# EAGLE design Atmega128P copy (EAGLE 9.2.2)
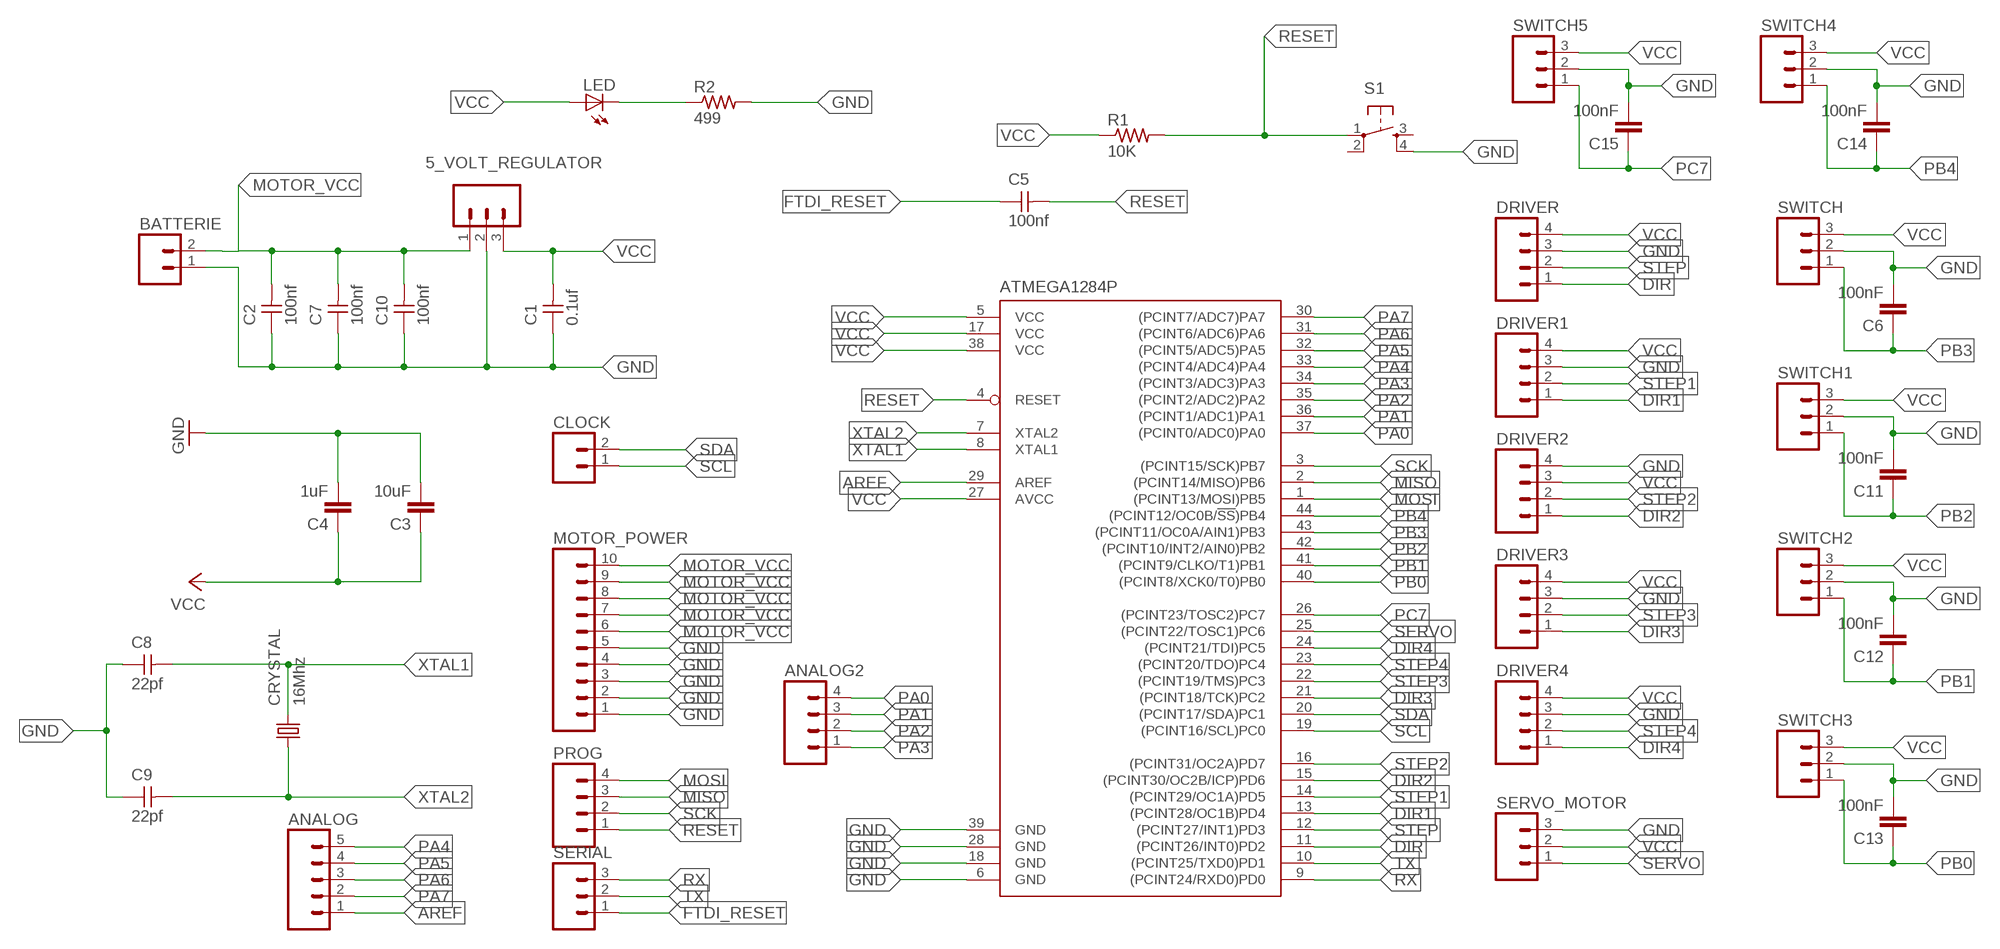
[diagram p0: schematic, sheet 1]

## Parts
5_VOLT_REGULATOR  M03  [03P]
ANALOG  M05  [05P]
ANALOG2  M04  [04P]
ATMEGA1284P  ATMEGA644A  [TQFP44]
BATTERIE  M02  [02P]
C1  0.1uf  UNPOLARIZED_CAPACITOR1206  [1206]
C2  100nf  UNPOLARIZED_CAPACITOR1206  [1206]
C3  10uF  CAP1206  [1206]
C4  1uF  CAP1206  [1206]
C5  100nf  UNPOLARIZED_CAPACITOR1206  [1206]
C6  100nF  CAP1206  [1206]
C7  100nf  UNPOLARIZED_CAPACITOR1206  [1206]
C8  22pf  UNPOLARIZED_CAPACITOR1206  [1206]
C9  22pf  UNPOLARIZED_CAPACITOR1206  [1206]
C10  100nf  UNPOLARIZED_CAPACITOR1206  [1206]
C11  100nF  CAP1206  [1206]
C12  100nF  CAP1206  [1206]
C13  100nF  CAP1206  [1206]
C14  100nF  CAP1206  [1206]
C15  100nF  CAP1206  [1206]
CLOCK  M02  [02P]
CRYSTAL  16Mhz  KX-12B  [6.0X3.5_2]
DRIVER  M04  [04P]
DRIVER1  M04  [04P]
DRIVER2  M04  [04P]
DRIVER3  M04  [04P]
DRIVER4  M04  [04P]
LED  LED1206  [1206]
MOTOR_POWER  M10  [10P]
PROG  M04  [04P]
R1  10K  RESISTOR1206  [1206]
R2  499  RESISTOR1206  [1206]
S1  6MM_SWITCH6MM_SWITCH  [6MM_SWITCH]
SERIAL  M03  [03P]
SERVO_MOTOR  M03  [03P]
SWITCH  M03  [03P]
SWITCH1  M03  [03P]
SWITCH2  M03  [03P]
SWITCH3  M03  [03P]
SWITCH4  M03  [03P]
SWITCH5  M03  [03P]

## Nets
AREF: ANALOG.1 ATMEGA1284P.29(AREF)
DIR: ATMEGA1284P.11((PCINT26/INT0)PD2) DRIVER.1
DIR1: ATMEGA1284P.13((PCINT28/OC1B)PD4) DRIVER1.1
DIR2: ATMEGA1284P.15((PCINT30/OC2B/ICP)PD6) DRIVER2.1
DIR3: ATMEGA1284P.21((PCINT18/TCK)PC2) DRIVER3.1
DIR4: ATMEGA1284P.24((PCINT21/TDI)PC5) DRIVER4.1
FTDI_RESET: C5.1 SERIAL.1
GND: 5_VOLT_REGULATOR.2 ATMEGA1284P.6(GND) ATMEGA1284P.18(GND) ATMEGA1284P.28(GND) ATMEGA1284P.39(GND) BATTERIE.1 C1.1 C2.1 C3.2 C4.2 C6.2 C7.1 C8.1 C9.1 C10.1 C11.2 C12.2 C13.2 C14.2 C15.2 DRIVER1.3 DRIVER2.4 DRIVER3.3 DRIVER4.3 DRIVER.3 MOTOR_POWER.1 MOTOR_POWER.2 MOTOR_POWER.3 MOTOR_POWER.4 MOTOR_POWER.5 R2.2 S1.4(S1) SERVO_MOTOR.3 SWITCH1.2 SWITCH2.2 SWITCH3.2 SWITCH4.2 SWITCH5.2 SWITCH.2
MISO: ATMEGA1284P.2((PCINT14/MISO)PB6) PROG.3
MOSI: ATMEGA1284P.1((PCINT13/MOSI)PB5) PROG.4
MOTOR_VCC: 5_VOLT_REGULATOR.1 BATTERIE.2 C2.2 C7.2 C10.2 MOTOR_POWER.6 MOTOR_POWER.7 MOTOR_POWER.8 MOTOR_POWER.9 MOTOR_POWER.10
N$1: LED.2(C) R2.1
PA0: ANALOG2.4 ATMEGA1284P.37((PCINT0/ADC0)PA0)
PA1: ANALOG2.3 ATMEGA1284P.36((PCINT1/ADC1)PA1)
PA2: ANALOG2.2 ATMEGA1284P.35((PCINT2/ADC2)PA2)
PA3: ANALOG2.1 ATMEGA1284P.34((PCINT3/ADC3)PA3)
PA4: ANALOG.5 ATMEGA1284P.33((PCINT4/ADC4)PA4)
PA5: ANALOG.4 ATMEGA1284P.32((PCINT5/ADC5)PA5)
PA6: ANALOG.3 ATMEGA1284P.31((PCINT6/ADC6)PA6)
PA7: ANALOG.2 ATMEGA1284P.30((PCINT7/ADC7)PA7)
PB0: ATMEGA1284P.40((PCINT8/XCK0/T0)PB0) C13.1 SWITCH3.1
PB1: ATMEGA1284P.41((PCINT9/CLKO/T1)PB1) C12.1 SWITCH2.1
PB2: ATMEGA1284P.42((PCINT10/INT2/AIN0)PB2) C11.1 SWITCH1.1
PB3: ATMEGA1284P.43((PCINT11/OC0A/AIN1)PB3) C6.1 SWITCH.1
PB4: ATMEGA1284P.44((PCINT12/OC0B/!SS!)PB4) C14.1 SWITCH4.1
PC7: ATMEGA1284P.26((PCINT23/TOSC2)PC7) C15.1 SWITCH5.1
RESET: ATMEGA1284P.4(RESET) C5.2 PROG.1 R1.2 S1.1(P)
RX: ATMEGA1284P.9((PCINT24/RXD0)PD0) SERIAL.3
SCK: ATMEGA1284P.3((PCINT15/SCK)PB7) PROG.2
SCL: ATMEGA1284P.19((PCINT16/SCL)PC0) CLOCK.1
SDA: ATMEGA1284P.20((PCINT17/SDA)PC1) CLOCK.2
SERVO: ATMEGA1284P.25((PCINT22/TOSC1)PC6) SERVO_MOTOR.1
STEP: ATMEGA1284P.12((PCINT27/INT1)PD3) DRIVER.2
STEP1: ATMEGA1284P.14((PCINT29/OC1A)PD5) DRIVER1.2
STEP2: ATMEGA1284P.16((PCINT31/OC2A)PD7) DRIVER2.2
STEP3: ATMEGA1284P.22((PCINT19/TMS)PC3) DRIVER3.2
STEP4: ATMEGA1284P.23((PCINT20/TDO)PC4) DRIVER4.2
TX: ATMEGA1284P.10((PCINT25/TXD0)PD1) SERIAL.2
VCC: 5_VOLT_REGULATOR.3 ATMEGA1284P.5(VCC) ATMEGA1284P.17(VCC) ATMEGA1284P.27(AVCC) ATMEGA1284P.38(VCC) C1.2 C3.1 C4.1 DRIVER1.4 DRIVER2.3 DRIVER3.4 DRIVER4.4 DRIVER.4 LED.1(A) R1.1 SERVO_MOTOR.2 SWITCH1.3 SWITCH2.3 SWITCH3.3 SWITCH4.3 SWITCH5.3 SWITCH.3
XTAL1: ATMEGA1284P.8(XTAL1) C8.2 CRYSTAL.2
XTAL2: ATMEGA1284P.7(XTAL2) C9.2 CRYSTAL.1
Unconnected: S1.2(P1) S1.3(S)

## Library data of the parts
5_VOLT_REGULATOR SERIAL SERVO_MOTOR SWITCH SWITCH1-SWITCH5 = con-amp-quick:M03: AMP QUICK CONNECTOR; OC_FARNELL: unknown; OC_NEWARK: unknown
ANALOG = con-amp-quick:M05: AMP QUICK CONNECTOR; OC_FARNELL: unknown; OC_NEWARK: unknown
ANALOG2 DRIVER DRIVER1-DRIVER4 PROG = con-amp-quick:M04: AMP QUICK CONNECTOR; OC_FARNELL: unknown; OC_NEWARK: unknown
ATMEGA1284P = atmel:ATMEGA644: 8-bit Microcontroller with 64K Bytes In-System Programmable Flash Source: http://www.atmel.com/dyn/resources/prod_documents/doc2593.pdf; MPN: ATMEGA644PV-10AU; OC_FARNELL: 1455123; OC_NEWARK: 58M3748
BATTERIE CLOCK = con-amp-quick:M02: AMP QUICK CONNECTOR; OC_FARNELL: unknown; OC_NEWARK: unknown
C1 C2 C5 C7-C10 = FAB_Hello:UNPOLARIZED_CAPACITOR: unpolarized_capacitor
C3 C4 C6 C11-C15 = 01_SparkFun:CAP: Capacitor
CRYSTAL = crystal-geyer_V1_0:KX
LED = FAB_Hello:LED
MOTOR_POWER = con-amp-quick:M10: AMP QUICK CONNECTOR; OC_FARNELL: unknown; OC_NEWARK: unknown
R1 R2 = FAB_Hello:RESISTOR
S1 = FAB_Hello:6MM_SWITCH: OMRON SWITCH

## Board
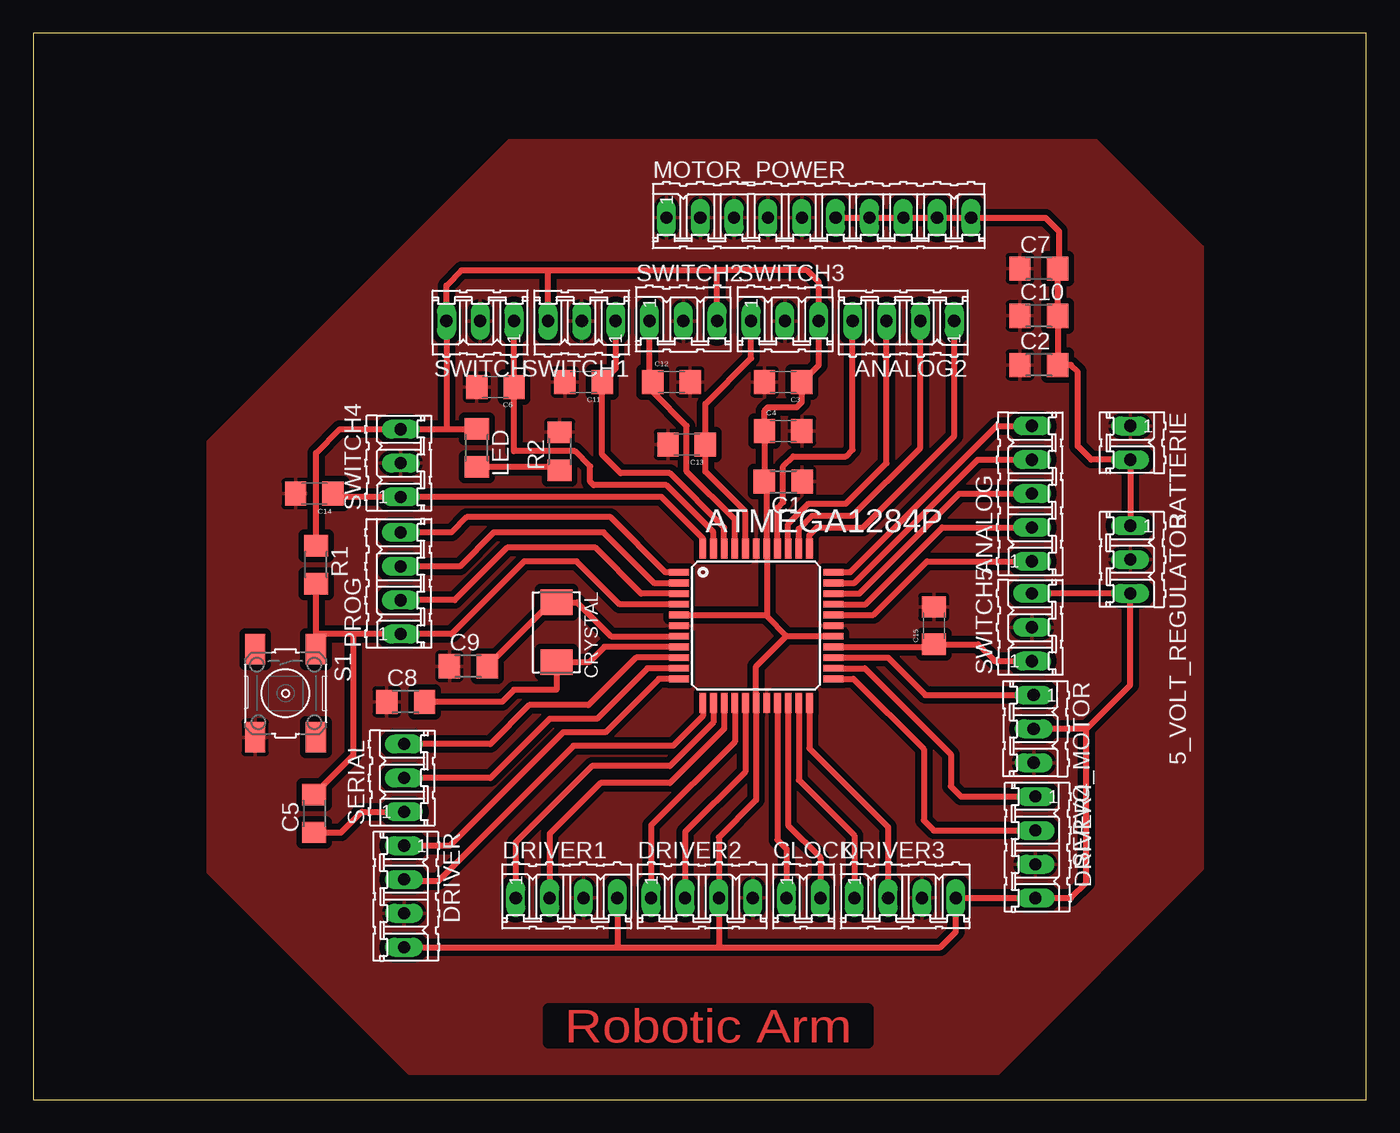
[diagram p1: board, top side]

Size 100 x 80 mm. Coordinates in mm from the lower left corner, seen from the top.
Outline: 0,0 100,0 100,80 0,80 0,0
Copper layers (1*16): Top 0.035mm / dielectric 1.5mm / Bottom 0.035mm
Design rules "default": minimum track width 6mil, minimum drill 0.35mm, track to track 6mil, track to pad 6mil, pad to pad 6mil, via to via 6mil, smd to smd 6mil, copper to edge 40mil, drill to drill 6mil, minimum pad ring 10mil, minimum via ring 8mil, stop-mask expansion 4mil, vias tented up to drill 0mil, thermal gap 10mil

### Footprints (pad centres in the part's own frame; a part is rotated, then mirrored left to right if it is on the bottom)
03P = drill 0.914 long: 1 -2.54,0; 2 0,0; 3 2.54,0
05P = drill 0.914 long: 1 -5.08,0; 2 -2.54,0; 3 0,0; 4 2.54,0; 5 5.08,0
04P = drill 0.914 long: 1 -3.81,0; 2 -1.27,0; 3 1.27,0; 4 3.81,0
TQFP44 = smd 1.5 x 0.5: 1 -5.8,4; 2 -5.8,3.2; 3 -5.8,2.4; 4 -5.8,1.6; 5 -5.8,0.8; 6 -5.8,0; 7 -5.8,-0.8; 8 -5.8,-1.6; 9 -5.8,-2.4; 10 -5.8,-3.2; 11 -5.8,-4; 23 5.8,-4; 24 5.8,-3.2; 25 5.8,-2.4; 26 5.8,-1.6; 27 5.8,-0.8; 28 5.8,0; 29 5.8,0.8; 30 5.8,1.6; 31 5.8,2.4; 32 5.8,3.2; 33 5.8,4 | smd 0.5 x 1.5: 12 -4,-5.8; 13 -3.2,-5.8; 14 -2.4,-5.8; 15 -1.6,-5.8; 16 -0.8,-5.8; 17 0,-5.8; 18 0.8,-5.8; 19 1.6,-5.8; 20 2.4,-5.8; 21 3.2,-5.8; 22 4,-5.8; 34 4,5.8; 35 3.2,5.8; 36 2.4,5.8; 37 1.6,5.8; 38 0.8,5.8; 39 0,5.8; 40 -0.8,5.8; 41 -1.6,5.8; 42 -2.4,5.8; 43 -3.2,5.8; 44 -4,5.8
02P = drill 0.914 long: 1 -1.27,0; 2 1.27,0
1206 = smd 1.6 x 1.803: 1 -1.422,0; 2 1.422,0
1206' = smd 1.6 x 1.8: 1 -1.4,0; 2 1.4,0
6.0X3.5_2 = smd 1.9 x 2.4: 1 -2.25,0; 2 2.25,0
10P = drill 0.914 long: 1 -11.43,0; 2 -8.89,0; 3 -6.35,0; 4 -3.81,0; 5 -1.27,0; 6 1.27,0; 7 3.81,0; 8 6.35,0; 9 8.89,0; 10 11.43,0
6MM_SWITCH = smd 2.286 x 1.524: 1 -3.302,2.286; 2 3.302,2.286; 3 -3.302,-2.286; 4 3.302,-2.286

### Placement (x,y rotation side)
5_VOLT_REGULATOR  82.3,40.51 270 top
ANALOG  74.93,45.47 90 top
ANALOG2  65.28,58.42 180 top
ATMEGA1284P  54.23,35.56 0 top
BATTERIE  82.3,49.28 270 top
C1  56.26,46.35 180 top
C2  75.44,55.12 0 top
C3  10uF  [1206']  56.26,53.85 180 top
C4  1uF  [1206']  56.26,50.16 0 top
C5  21.08,21.46 90 top
C6  100nF  [1206']  34.67,53.47 180 top
C7  75.44,62.36 0 top
C8  27.94,29.84 0 top
C9  32.64,32.51 0 top
C10  75.44,58.8 0 top
C11  100nF  [1206']  41.27,53.85 180 top
C12  100nF  [1206']  47.88,53.85 0 top
C13  100nF  [1206']  49.02,49.15 180 top
C14  100nF  [1206']  21.08,45.47 180 top
C15  100nF  [1206']  67.56,35.56 90 top
CLOCK  57.78,15.11 0 top
CRYSTAL  39.24,35.05 270 top
DRIVER  27.81,15.24 270 top
DRIVER1  40.01,15.11 0 top
DRIVER2  50.16,15.11 0 top
DRIVER3  65.41,15.11 0 top
DRIVER4  75.18,18.92 270 top
LED  33.27,48.9 270 top
MOTOR_POWER  58.93,66.17 0 top
PROG  27.56,38.73 90 top
R1  21.21,40.13 270 top
R2  39.5,48.64 90 top
S1  18.92,30.48 270 top
SERIAL  27.81,24.13 90 top
SERVO_MOTOR  75.06,27.81 270 top
SWITCH  33.53,58.42 180 top
SWITCH1  41.15,58.42 180 top
SWITCH2  48.77,58.42 0 top
SWITCH3  56.39,58.42 0 top
SWITCH4  27.56,47.75 90 top
SWITCH5  74.93,35.43 90 top

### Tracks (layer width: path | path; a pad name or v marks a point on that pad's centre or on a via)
AREF
  Top 0.432: ATMEGA1284P.29 63.03,36.36 67.06,40.39 ANALOG.1
DIR
  Top 0.432: ATMEGA1284P.11 46.93,31.56 42.93,27.56 39.75,27.56 31.24,19.05 DRIVER.1
DIR1
  Top 0.432: ATMEGA1284P.13 51.03,28.3 47.75,25.02 41.91,25.02 36.2,19.3 DRIVER1.1
DIR2
  Top 0.432: ATMEGA1284P.15 52.63,26.85 46.35,20.57 DRIVER2.1
DIR3
  Top 0.432: ATMEGA1284P.21 57.43,23.98 61.59,19.81 DRIVER3.1
DIR4
  Top 0.432: ATMEGA1284P.24 62.38,32.36 68.83,25.91 68.83,23.5 69.6,22.73 DRIVER4.1
FTDI_RESET
  Top 0.432: C5.1 23.09,20.04 23.81,20.77 24.64,21.59 SERIAL.1
GND
  pour Top (isolate 0.432): 35.69,72.01 79.76,72.01 87.76,64.01 87.76,17.27 72.39,1.91 28.19,1.91 13.08,17.02 13.08,49.4
MISO
  Top 0.432: ATMEGA1284P.2 48.4,38.73 46.61,38.73 42.8,42.55 34.54,42.55 32,40.01 PROG.3
MOSI
  Top 0.432: ATMEGA1284P.1 47.44,39.56 43.31,43.69 32.51,43.69 31.37,42.55 PROG.4
MOTOR_VCC
  Top 0.432: MOTOR_POWER.6 MOTOR_POWER.7 MOTOR_POWER.8 MOTOR_POWER.9 MOTOR_POWER.10 75.95,66.17 76.96,65.15 76.96,62.08 76.86,61.98 | 5_VOLT_REGULATOR.1 BATTERIE.2 79.38,48.01 78.36,49.02 78.36,54.61 77.85,55.12 C2.2 C10.2 76.86,61.98 | 76.86,61.98 C7.2
N$1
  Top 0.432: R2.1 39.24,47.47 LED.2
PA0
  Top 0.432: ATMEGA1284P.37 55.83,44.4 56.26,44.83 56.26,47.5 57.02,48.26 60.96,48.26 61.47,48.77 ANALOG2.4
PA1
  Top 0.432: ATMEGA1284P.36 56.63,43.17 58.17,44.7 60.96,44.7 64.01,47.75 ANALOG2.3
PA2
  Top 0.432: ATMEGA1284P.35 57.43,42.82 58.42,43.81 61.47,43.81 66.55,48.9 ANALOG2.2
PA3
  Top 0.432: ATMEGA1284P.34 58.23,42.35 58.8,42.93 62.23,42.93 69.09,49.78 ANALOG2.1
PA4
  Top 0.432: ANALOG.5 72.26,50.55 61.34,39.62 61.28,39.56 ATMEGA1284P.33
PA5
  Top 0.432: ATMEGA1284P.32 61.62,38.76 70.87,48.01 ANALOG.4
PA6
  Top 0.432: ATMEGA1284P.31 61.96,37.96 69.47,45.47 ANALOG.3
PA7
  Top 0.432: ATMEGA1284P.30 62.43,37.16 68.2,42.93 ANALOG.2
PB0
  Top 0.432: ATMEGA1284P.40 53.43,44.11 50.42,47.12 C13.1 50.42,52.2 53.85,55.63 SWITCH3.1
PB1
  Top 0.432: ATMEGA1284P.41 52.63,43.51 49.02,47.12 49.02,50.55 46.48,53.09 C12.1 46.23,54.1 SWITCH2.1
PB2
  Top 0.432: ATMEGA1284P.42 51.83,42.91 47.75,46.99 44.07,46.99 42.67,48.38 C11.1 43.69,54.86 SWITCH1.1
PB3
  Top 0.432: ATMEGA1284P.43 51.03,42.57 47.5,46.1 42.04,46.1 41.78,46.35 41.78,47.5 40.64,48.64 36.07,48.64 C6.1 SWITCH.1
PB4
  Top 0.432: ATMEGA1284P.44 50.23,42.1 47.12,45.21 SWITCH4.1 22.74,45.21 C14.1
PC7
  Top 0.432: ATMEGA1284P.26 67.36,33.96 C15.1 70.87,34.16 72.14,32.89 SWITCH5.1
RESET
  Top 0.432: 24,34.92 PROG.1 31.37,34.92 36.83,40.39 40.77,40.39 43.99,37.16 ATMEGA1284P.4 | 24,34.92 21.34,34.92 21.21,34.8 | S1.1 R1.2 | 24,34.92 24,25.81 C5.2
  Top 0.457: S1.1 21.21,34.8
RX
  Top 0.432: ATMEGA1284P.9 45.23,33.16 41.66,29.59 37.21,29.59 34.29,26.67 SERIAL.3
SCK
  Top 0.432: ATMEGA1284P.3 45.61,37.96 42.16,41.4 35.56,41.4 31.62,37.47 PROG.2
SCL
  Top 0.432: ATMEGA1284P.19 55.83,19.48 56.52,18.8 CLOCK.1
SDA
  Top 0.432: ATMEGA1284P.20 56.63,20.59 59.05,18.16 CLOCK.2
SERVO
  Top 0.432: ATMEGA1284P.25 64.12,33.16 66.93,30.35 SERVO_MOTOR.1
STEP
  Top 0.432: ATMEGA1284P.12 50.23,28.77 48.01,26.54 40.51,26.54 30.35,16.38 27.94,16.38 DRIVER.2
STEP1
  Top 0.432: DRIVER1.2 38.73,19.94 42.55,23.75 47.75,23.75 51.82,27.81 51.83,27.83 ATMEGA1284P.14
STEP2
  Top 0.432: ATMEGA1284P.16 53.43,24.6 48.9,20.07 DRIVER2.2
STEP3
  Top 0.432: ATMEGA1284P.22 58.23,26.35 64.14,20.45 DRIVER3.2
STEP4
  Top 0.432: ATMEGA1284P.23 61.53,31.56 66.8,26.29 66.8,20.95 67.56,20.19 DRIVER4.2
TX
  Top 0.432: ATMEGA1284P.10 46.08,32.36 42.29,28.57 38.73,28.57 34.29,24.13 SERIAL.2
VCC
  Top 0.432: SWITCH5.3 5_VOLT_REGULATOR.3 82.3,31.11 78.99,27.81 | 51.44,11.43 68.07,11.43 69.22,12.57 DRIVER3.4 DRIVER4.4 77.85,15.11 78.99,16.26 78.99,27.81 | 51.44,11.43 DRIVER2.3 51.44,19.68 54.23,22.48 ATMEGA1284P.17 54.23,32.51 56.52,34.8 | 78.99,27.81 SERVO_MOTOR.2 | 56.52,34.8 59.99,34.8 ATMEGA1284P.27 | 54.86,46.5 C4.1 54.86,51.69 55.12,51.94 57.28,51.94 57.66,52.33 C3.1 58.93,55.12 SWITCH3.3 58.93,61.34 58.04,62.23 51.31,62.23 | 54.86,46.5 54.86,46.38 C1.2 | 54.86,46.5 55.03,46.34 ATMEGA1284P.38 55.03,36.32 | DRIVER.4 43.81,11.43 | 43.81,11.43 51.44,11.43 | R1.1 21.21,48.51 22.99,50.29 SWITCH4.3 30.99,50.29 | 30.99,50.29 SWITCH.3 30.99,61.09 32.13,62.23 38.61,62.23 | 38.61,62.23 51.31,62.23 | SWITCH2.3 51.31,62.23 | SWITCH1.3 38.61,62.23 | 55.03,36.32 55.03,36.28 56.52,34.8 | ATMEGA1284P.5 54.99,36.36 55.03,36.32 | 30.99,50.29 33.25,50.29 LED.1 | DRIVER1.4 43.81,11.43
XTAL1
  Top 0.432: ATMEGA1284P.8 42.85,33.96 41.69,32.8 CRYSTAL.2 39.24,30.73 36.07,30.73 35.18,29.84 C8.2
XTAL2
  Top 0.432: C9.2 38.85,37.3 CRYSTAL.1 40.8,37.3 43.34,34.76 ATMEGA1284P.7

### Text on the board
Top: Robotic Arm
